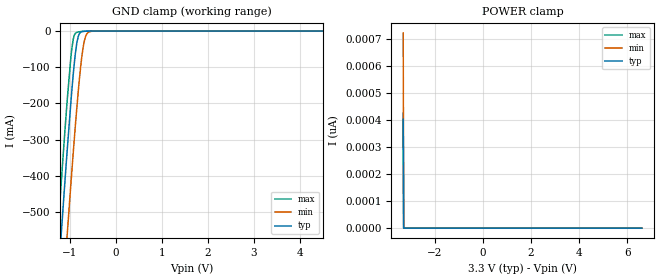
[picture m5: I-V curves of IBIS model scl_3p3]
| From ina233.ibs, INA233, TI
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|   scl_3p3
[Model]   scl_3p3
Model_type   Input
Vinl = 0.4
Vinh = 2.31
|   typ   min   max
C_comp   6.147E-13   5.919E-13   6.360E-13
| Where Nom  PVT is Nominal Process, 3.3V, 25C
|   Fast PVT is Strong Process,  3.6V, -40C
|   Slow PVT is Weak Process,   2.7V, 125C
[Voltage Range]   3.3   2.7   3.6
[Temperature Range]   25   125   -40
[Power Clamp Reference]   3.3   2.7   3.6
[GND Clamp Reference]   0   0   0
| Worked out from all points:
|   GND clamp passes 1 mA (typ) near -0.71 V on its own axis
[GND Clamp]
|   Voltage   I(typ)   I(min)   I(max)
-3.3V     -4.686A    -4.907A    -4.556A
-1.251V   -685.9mA   -923.4mA   -543.4mA
-1.181V   -558mA     -795.1mA   -415.7mA
-1.053V   -328.1mA   -561.6mA   -190.2mA
-953.7mV  -165.6mA   -388.9mA   -49.35mA
-904.2mV  -95.52mA   -306.4mA   -13.32mA
-844.8mV  -33.22mA   -212.7mA   -3.47mA
-765.6mV  -3.856mA   -104mA     -1.449mA
-696.3mV  -740.9uA   -37.2mA    -647.4uA
-636.9mV  -214.4uA   -10.28mA   -278.8uA
-547.8mV  -30.3uA    -1.138mA   -47.56uA
6.6V      0A         0A         0A
[POWER Clamp]
|   Voltage   I(typ)   I(min)   I(max)
-3.3V     402.2pA    721.3pA    425.3pA
-3.28V    0A         0A         0A
-3.27V    0A         0A         0A
6.6V      0A         0A         0A
